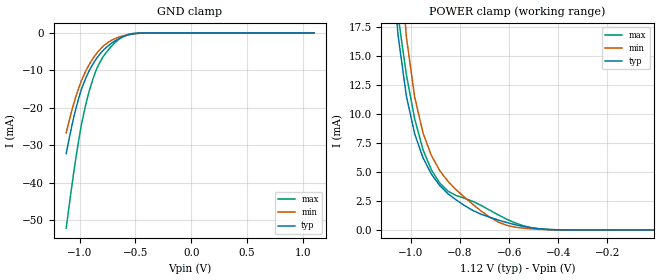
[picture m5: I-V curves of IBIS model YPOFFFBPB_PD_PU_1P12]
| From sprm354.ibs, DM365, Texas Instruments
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|   Model Cell YPOFFFBPB_PD_PU_1P12
|BQ1865ACTHYPOFFFBPB_PD_PU_1P12
[Model]   YPOFFFBPB_PD_PU_1P12
Model_type   Input
Polarity   Non-Inverting
Vinl =  0.392V
Vinh =  0.728V
C_comp   0.683176p   0.4871003p   1.466367p
[Model Spec]
Vinl   0.392   0.35   0.43050
Vinh   0.728   0.65   0.79950
[Temperature Range]   25   125   -40
[Voltage Range]   1.12   1   1.23
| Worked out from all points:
|   GND clamp passes 1 mA (typ) near -0.61 V on its own axis
|   POWER clamp passes 1 mA (typ) near -0.67 V on its own axis
[POWER_clamp]
|   voltage   I(typ)   I(min)   I(max)
-1.12V    41.71mA    68.47mA    36.86mA
-1.052V   16.79mA    25.68mA    18.5mA
-1.041V   15.04mA    22.66mA    16.79mA
-1.018V   11.54mA    16.64mA    13.38mA
-984.2mV  8.28mA     11.44mA    9.564mA
-950.3mV  6.201mA    8.35mA     6.908mA
-882.4mV  3.828mA    5.114mA    4.044mA
-814.5mV  2.577mA    3.445mA    2.958mA
-678.8mV  1.092mA    1.098mA    1.704mA
-577mV    459uA      246.1uA    621.6uA
-441.2mV  49.72uA    32.54uA    30.31uA
-11.31mV  205.9pA    2.566nA    47.56pA
[GND_clamp]
|   voltage   I(typ)   I(min)   I(max)
-1.12V    -32.22mA   -26.7mA    -52.14mA
-1.052V   -22.46mA   -18.81mA   -37.12mA
-1.007V   -17.35mA   -14.64mA   -28.48mA
-961.6mV  -13.31mA   -11.26mA   -21.34mA
-916.4mV  -10.21mA   -8.547mA   -15.76mA
-848.5mV  -6.83mA    -5.489mA   -9.653mA
-803.2mV  -5.139mA   -3.975mA   -7.047mA
-712.7mV  -2.72mA    -1.933mA   -3.488mA
-644.8mV  -1.494mA   -1.086mA   -1.631mA
-577mV    -649.1uA   -547uA     -509.6uA
-463.8mV  -79.77uA   -107.3uA   -40.96uA
1.097V    163.1pA    14.04nA    40.22pA
